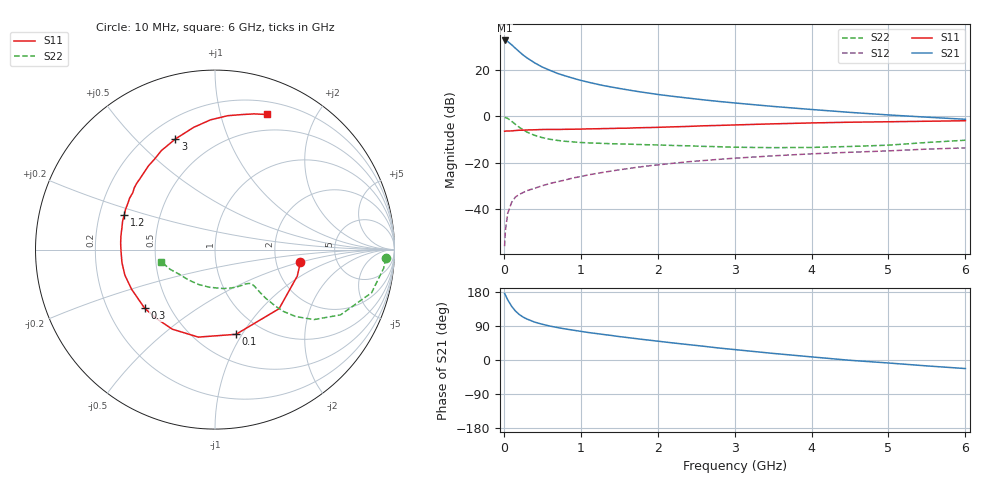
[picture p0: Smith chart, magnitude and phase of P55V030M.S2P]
! SIEMENS Small Signal Semiconductors
! BFP183
! Si NPN RF Bipolar Junction Transistor in SOT143
! VCE = 5 V  IC = 30 mA
! Common Emitter S-Parameters:  March  1996
# GHz  S  MA  R  50
!  f  S11  S21  S12  S22
! GHz  MAG  ANG  MAG  ANG  MAG  ANG  MAG  ANG
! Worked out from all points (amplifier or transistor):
!   36 points, 10 MHz to 6 GHz, reference 50 ohm
!   highest |S21| = 32.7 dB at 10 MHz (marker M1)
!   |S21| within 3 dB of that: start of sweep to 138.8 MHz
!   unconditionally stable (mu >= 1): 692.4 MHz to 5.688 GHz
!   at 250 MHz: K = 0.57, MSG = 29.6 dB, |S12| = -32.8 dB
!   at 1.4 GHz: K = 1.15, MAG = 15.8 dB, |S12| = -23.5 dB
!   at 6 GHz: K = 0.97, MSG = 6.2 dB, |S12| = -13.6 dB
!   S11 on the Smith chart (normalised r, x): 10 MHz: 2.74, -0.51; 100 MHz: 0.76, -0.94; 300 MHz: 0.36, -0.32; 1.2 GHz: 0.31, +0.17; 3 GHz: 0.31, +0.66; 6 GHz: 0.33, +1.40
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0.01  0.4807 -8.5  43.26 175.4  0.0016 85.7  0.9533 -2.9
0.02  0.4816 -17.8  43.17 171.4  0.0034 84.2  0.9454 -6.3
0.05  0.4857 -42.7  41.06 159.0  0.0081 78.2  0.9049 -15.4
0.1  0.4863 -76.1  35.08 142.1  0.0139 62.8  0.7881 -27.5
0.15  0.4963 -100.8  29.46 129.4  0.0183 56.6  0.6748 -35.3
0.2  0.5032 -118.2  24.81 120.2  0.0208 54.5  0.5835 -39.7
0.25  0.5043 -130.9  21.05 113.3  0.0229 51.9  0.5137 -42.1
0.3  0.5101 -140.3  18.25 108.2  0.0251 51.6  0.4596 -43.1
0.4  0.5146 -154.6  14.26 100.0  0.0283 51.8  0.3907 -43.8
0.5  0.522 -164.2  11.57 94.3  0.0321 52.1  0.3488 -43.6
0.6  0.5235 -172.1  9.816 89.5  0.0359 53.7  0.3215 -43.2
0.7  0.5234 -178.4  8.414 85.5  0.0392 54.8  0.3033 -42.9
0.8  0.5269 176.1  7.444 81.9  0.0427 55.3  0.2906 -42.9
1.1  0.5387 162.8  5.45 72.5  0.055 56.8  0.2686 -44.5
1.2  0.5411 158.9  4.991 69.9  0.0587 56.3  0.265 -45.4
1.7  0.5665 142.5  3.523 56.9  0.0787 54.1  0.2501 -52.6
2.2  0.5956 128.6  2.704 45.0  0.0977 50.2  0.2366 -62.5
3  0.6547 109.7  1.948 27.5  0.1256 42.9  0.2168 -83.1
3.5  0.691 100.0  1.641 17.4  0.1413 38.3  0.2121 -98.4
4.5  0.7493 84.6  1.221 -0.8  0.1688 28.9  0.2249 -131.4
5.5  0.7862 74.1  0.962 -15.6  0.1975 21.0  0.2742 -156.6
6  0.8059 69.1  0.867 -22.6  0.2098 16.4  0.3069 -167.3
